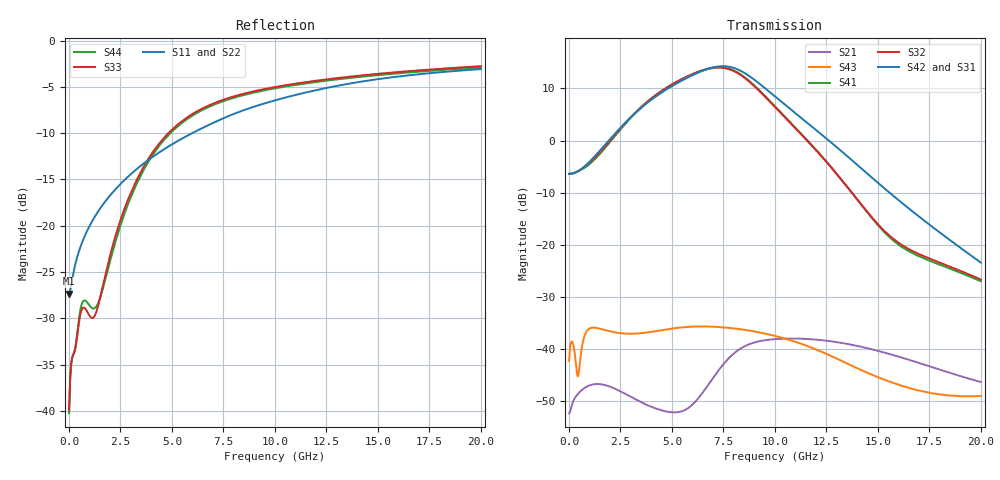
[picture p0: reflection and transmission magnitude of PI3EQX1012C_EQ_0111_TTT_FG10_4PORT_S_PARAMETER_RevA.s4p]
! NPort=4 DATA=2000 NOISE=0 GROUPDELAY=0 COMPLEX_DATAFORMAT=POLAR
! NumOfBlock=1 NumOfParam=0
! .MODEL Smodel S TSTONEFILE=PI3EQX1012C_EQ_0111_TTT_FG10_4PORT_S_PARAMETER_RevA.s4p TYPE=S
!  -- The above .MODEL line can be used for the S element in the netlist.
! The s parameter is extracted from the linear redriver, it is not bi-directional; only s(4,1)s(4,2) and s(3,1)s(3,2)
! should be the insertion loss
!Port definition:
!Port1 = input+
!Port2 = input-
!Port3 = output+
!Port4 = output-
# Hz S MA R  50
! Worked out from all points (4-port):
!   2000 points, 10 MHz to 20 GHz, reference 50 ohm
!   strongest paths, dB at 10 MHz, 5.01 GHz, 10.01 GHz, 15.01 GHz, 20 GHz:
!     S42: -6.4, 10.5, 8.4, -8.2, -23.5
!     S31: -6.4, 10.5, 8.4, -8.4, -23.9
!     S32: -6.4, 10.8, 6.4, -16.1, -26.7
!     S41: -6.4, 10.8, 6.6, -16.3, -27.1
!     S43: -42.4, -36.2, -37.6, -45.5, -49.1
!     S21: -52.4, -52.2, -38.2, -40.4, -46.4
!   lowest |S11| = -27.3 dB at 10 MHz (marker M1), VSWR 1.09, Z = 45.9 - j0.123 ohm
!   |S11| at or under -10 dB: start of sweep to 5.985 GHz
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1e7  0.04301 -178.2  0.002379 1.5  0.0008102 -0.5  0.0008039 -0.5
     0.002388 1.5  0.04109 -178.1  0.000927 -0.5  0.0009197 -0.5
     0.4784 -0.1  0.4775 180.0  0.01016 -4.0  0.007598 -25.7
     0.4771 180.0  0.4794 -0.1  0.007615 -25.8  0.009722 -4.0
4.1e9  0.2369 -124.3  0.002739 0.1  0.0003815 -56.8  0.0003797 -57.2
       0.002711 0.3  0.2405 -123.2  0.0004336 -57.5  0.0004316 -57.9
       2.55 -62.3  2.63 127.9  0.2524 -83.6  0.0136 33.7
       2.615 128.6  2.548 -60.6  0.01458 30.7  0.2445 -83.3
5.72e9  0.3051 -123.8  0.002685 39.9  0.0002788 -58.4  0.0002777 -59.3
        0.002626 38.2  0.3101 -123.1  0.0003162 -59.3  0.000315 -60.2
        3.967 -129.1  4.094 60.7  0.3833 -99.2  0.01637 9.9
        4.108 61.0  3.984 -127.2  0.01614 7.2  0.3755 -99.0
7.01e9  0.3596 -124.4  0.005514 59.3  0.0002404 -55.9  0.0002384 -57.3
        0.005265 59.7  0.3651 -123.9  0.0002712 -57.1  0.000269 -58.5
        5.016 167.2  4.977 -3.4  0.457 -109.3  0.01672 -10.2
        5.018 -3.5  5.047 169.3  0.01623 -11.2  0.4488 -109.1
8.14e9  0.407 -125.8  0.009687 42.7  0.0002243 -54.2  0.0002212 -55.7
        0.009412 44.0  0.413 -125.3  0.0002514 -55.5  0.0002481 -57.0
        4.838 102.5  4.505 -68.0  0.5041 -116.1  0.01588 -25.7
        4.558 -68.5  4.871 104.9  0.01553 -26.1  0.4956 -115.9
9.49e9  0.4575 -128.1  0.01218 15.0  0.0002143 -53.9  0.0002102 -55.4
        0.01201 16.3  0.4644 -127.6  0.0002384 -55.0  0.0002341 -56.6
        3.194 33.5  2.674 -135.6  0.5472 -122.2  0.01427 -41.9
        2.715 -136.6  3.219 36.2  0.01398 -42.4  0.5384 -122.1
2e10  0.7011 -144.6  0.004833 -71.4  0.0001465 -72.3  0.0001413 -73.8
      0.004778 -70.7  0.7161 -144.4  0.0001624 -72.1  0.0001567 -73.8
      0.06377 105.2  0.04609 31.6  0.7272 -143.5  0.003581 -51.6
      0.04433 29.9  0.06705 110.0  0.0035 -48.9  0.7152 -143.3
